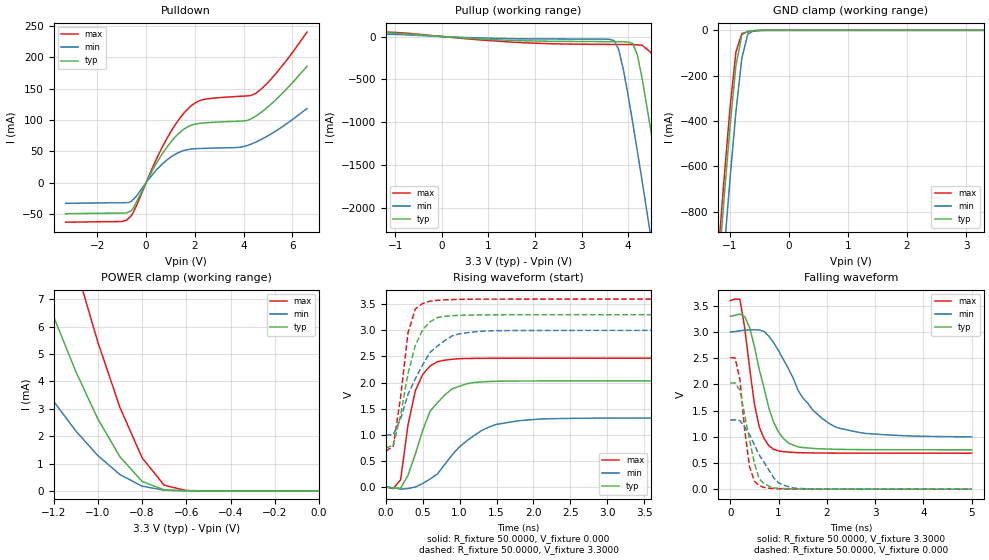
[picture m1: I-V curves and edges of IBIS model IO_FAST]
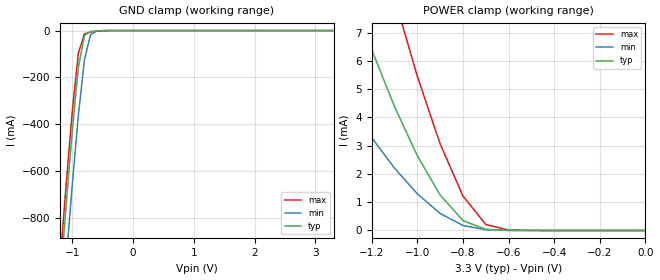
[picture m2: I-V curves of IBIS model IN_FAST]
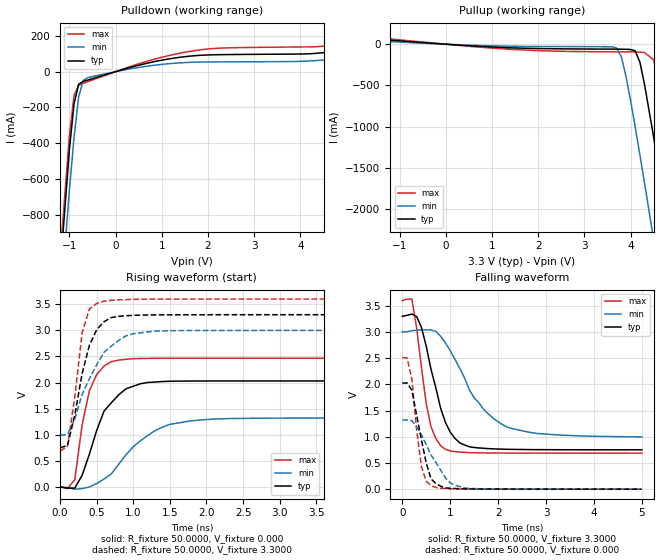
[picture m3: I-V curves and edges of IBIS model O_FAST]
| IBIS file xc4kxl.ibs created by s2ibis2 version 1.1
| North Carolina State University Electronics Research Laboratory  1995
[IBIS ver]   2.1
[File name]   xc4kxl.ibs
[File Rev]   1.5
[Date]   June 18, 2002
[Source]   Hspice simulations (35sTT,SS,FF)
[Notes]   Xilinx IBIS model for XC4kxl (fast slew rate)
   The package models are provided for BG432, BG256, BG352,
   BG560, HQ240, HT144, PQ240, PQ208, PQ160, PQ100, TQ144,
   and VQ100 package types, with BG432 as default. Please make
   your own selection of the packages by commenting out those
   unused ones.
   Control flag setting:
   2 slew rate opts are provided in the model: fast and slow.
   IO_FAST - Input/output Buffer model & fast slew rate
   I_FAST  - Input Buffer model & fast slew rate
   O_FAST  - Output Buffer model & fast slew rate
   IO_SLOW - Input/output Buffer model & slow slew rate
   I_SLOW  - Input Buffer model & slow slew rate
   O_SLOW  - Output Buffer model & slow slew rate
   COMMENTS: Models include process corners for MIN and MAX.
[Disclaimer] The data in this model is derived from SPICE simulations using
   modeling information extracted from the target process. While
   a great deal of care has been taken to provide information
   that is accurate, this model is considered preliminary as it
   has not been verified by actual silicon measurement. Treat the
   data in this model as preliminary until actual silicon
   verification is performed.
[Copyright]   Copyright 2002, Xilinx Inc., All rights reserved
|   Component XC4kxl
|   >>> Make Your Selection of the Package type Below <<<
[Component]   XC4kxl
[Manufacturer]   Xilinx Inc.
[Package]
| For package type BG432
| variable   typ   min   max
R_pkg   0.2500   0.1600   0.3500
L_pkg   4.9000nH   2.4000nH   7.4000nH
C_pkg   1.1500pF   0.8000pF   1.5000pF
| For package type BG256
| variable   typ   min   max
|R_pkg   0.057   0.05   0.065
|L_pkg   4.65nH   3.30nH   6.00nH
|C_pkg   1.05pF   0.80pF   1.30pF
| For package type BG352
| variable   typ   min   max
|R_pkg   0.218   0.145   0.290
|L_pkg   7.20nH   3.40nH   11.0nH
|C_pkg   0.95pF   0.70pF   1.20pF
| For package type BG560
| variable   typ   min   max
|R_pkg   0.24   0.16   0.32
|L_pkg   6.05nH   3.90nH   8.20nH
|C_pkg   1.05pF   0.70pF   1.40pF
| For package type HQ240
| variable   typ   min   max
|R_pkg   0.208   0.202   0.215
|L_pkg   13.2nH   9.00nH   17.3nH
|C_pkg   2.60pF   2.00pF   3.20pF
| For package type HT144
| variable   typ   min   max
|R_pkg   0.115   0.105   0.124
|L_pkg   9.05nH   4.80nH   13.3nH
|C_pkg   0.90pF   0.70pF   1.10pF
| For package type PQ240
| variable   typ   min   max
|R_pkg   0.208   0.205   0.218
|L_pkg   18.9nH   11.9nH   25.8nH
|C_pkg   2.00pF   1.30pF   2.70pF
| For package type PQ208
| variable   typ   min   max
|R_pkg   0.160   0.120   0.200
|L_pkg   18.7nH   10.3nH   27.0nH
|C_pkg   1.80pF   0.70pF   2.90pF
| For package type PQ160
| variable   typ   min   max
|R_pkg   0.195   0.18   0.21
|L_pkg   18.5nH   11.3nH   25.6nH
|C_pkg   2.10pF   1.50pF   2.70pF
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[Pin]  signal_name   model_name   R_pin   L_pin   C_pin
1   IO_FAST   IO_FAST
1I   I_FAST   IN_FAST
1O   O_FAST   O_FAST
2   IO_SLOW   IO_SLOW
2I   I_SLOW   IN_SLOW
2O   O_SLOW   O_SLOW
3   gnd   GND
4   vdd   POWER
| Models and submodels in the file (6): IO_FAST (I/O), IN_FAST (Input), O_FAST (Output), IO_SLOW (I/O), IN_SLOW (Input), O_SLOW (Output)
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|   Model IO_FAST
[Model]   IO_FAST
Model_type   I/O
Polarity   Non-Inverting
Enable   Active-Low
Vmeas =   1.6500V
Vinl =  0.8
Vinh =  2.0
Cref =  50.0000pF
Rref =   1.0000M
Vref =  0.000V
C_comp   7.0000pF   6.0000pF   8.0000pF
[Temperature Range]   27.0000   100.0000   0.000
[Voltage Range]   3.3000V   3.0000V   3.6000V
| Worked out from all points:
|   slope of the pulldown table from 0 to 0.495 V, typ, clamps not added: 13.9 ohm
|   slope of the pullup table from 0 to 0.495 V, typ, clamps not added: 27.1 ohm
|   GND clamp passes 1 mA (typ) near -0.58 V on its own axis
|   POWER clamp passes 1 mA (typ) near -0.87 V on its own axis
|   rising waveform, R_fixture 50.0000, V_fixture 0.000: 20-80 % time 362ps typ, 565ps min, 207ps max; typ from 0 V to 2.03 V
|   rising waveform, R_fixture 50.0000, V_fixture 3.3000: 20-80 % time 245ps typ, 395ps min, 162ps max; typ from 0.751 V to 3.3 V
|   falling waveform, R_fixture 50.0000, V_fixture 3.3000: 20-80 % time 425ps typ, 818ps min, 274ps max; typ from 3.3 V to 0.751 V
|   falling waveform, R_fixture 50.0000, V_fixture 0.000: 20-80 % time 275ps typ, 478ps min, 180ps max; typ from 2.02 V to 0.001 V
[Pulldown]
| voltage   I(typ)   I(min)   I(max)
-3.3V     -49.3mA    -32.8mA    -62.8mA
-800mV    -48.11mA   -31.6mA    -59.6mA
-500mV    -38.84mA   -25.82mA   -45.39mA
300mV     22.39mA    14.76mA    27.1mA
800mV     53.74mA    34.43mA    66.56mA
1.3V      76.97mA    47.48mA    98.21mA
1.7V      88.86mA    52.78mA    117.1mA
2.3V      95.03mA    54.68mA    131.9mA
3.8V      98.02mA    56.26mA    137.5mA
4.5V      106mA      64.68mA    142.4mA
5.3V      131.4mA    81.93mA    172.8mA
6.6V      185.5mA    118.2mA    239.9mA
[Pullup]
| voltage   I(typ)   I(min)   I(max)
-3.3V     63.98mA    45.77mA    74.9mA
3.7V      -59.9mA    -48.13mA   -92.59mA
3.8V      -60.3mA    -155.1mA   -92.88mA
3.9V      -61.55mA   -391.7mA   -93.16mA
4.1V      -81.44mA   -1.009A    -94.6mA
4.2V      -218.1mA   -1.343A    -97.2mA
4.3V      -487mA     -1.684A    -101mA
4.5V      -1.135A    -2.381A    -191.2mA
4.7V      -1.825A    -3.088A    -749.8mA
4.9V      -2.532A    -3.801A    -1.425A
5.1V      -3.246A    -4.519A    -2.126A
6.6V      -8.69A     -9.964A    -7.553A
[GND_clamp]
| voltage   I(typ)   I(min)   I(max)
-3.3V     -8.626A    -8.837A    -8.551A
-1.2V     -1.073A    -1.312A    -987.3mA
-1.1V     -740.8mA   -978.2mA   -654.8mA
-1V       -426mA     -657.1mA   -343.9mA
-900mV    -157.2mA   -360.9mA   -96.62mA
-800mV    -20.77mA   -124.4mA   -14.17mA
-700mV    -3.846mA   -17.61mA   -6.82mA
-600mV    -1.246mA   -1.662mA   -3.283mA
-300mV    -276.3nA   -435.5nA   -2.755uA
3.3V      151.6pA    7.389nA    160.4pA
[POWER_clamp]
| voltage   I(typ)   I(min)   I(max)
-3.3V     75.42mA    47.28mA    100.2mA
-1.5V     13.67mA    7.363mA    21.72mA
-1.4V     11.06mA    5.873mA    18.06mA
-1.3V     8.626mA    4.508mA    14.56mA
-1.2V     6.385mA    3.279mA    11.27mA
-1.1V     4.373mA    2.199mA    8.21mA
-1V       2.636mA    1.293mA    5.443mA
-900mV    1.25mA     599.1uA    3.055mA
-800mV    347.4uA    174.4uA    1.214mA
-700mV    37.68uA    27.06uA    209.3uA
-600mV    2.828uA    3.397uA    13.73uA
0V        151.6pA    186pA      177.1pA
[Ramp]
| variable   typ   min   max
dV/dt_r   1.1778/0.3241n   0.7476/0.5583n   1.4796/0.2068n
dV/dt_f   1.5292/0.3940n   1.2009/0.8182n   1.7477/0.2630n
R_load = 50.0000
[Rising Waveform]
R_fixture = 50.0000
V_fixture = 0.000
| time   V(typ)   V(min)   V(max)
0s        0V         0V         0V
100ps     -22.13mV   -13.9mV    -32.02mV
200ps     -22.59mV   -42.96mV   137.3mV
300ps     222.1mV    -31.55mV   1.186V
400ps     629.5mV    -1.35mV    1.845V
600ps     1.453V     151.4mV    2.316V
700ps     1.614V     249.8mV    2.4V
1ns       1.93V      771.6mV    2.457V
1.5ns     2.025V     1.199V     2.465V
5ns       2.03V      1.32V      2.466V
[Rising Waveform]
R_fixture = 50.0000
V_fixture = 3.3000
V_fixture_min = 3.0000
V_fixture_max = 3.6000
| time   V(typ)   V(min)   V(max)
0s        750.6mV    990.1mV    686.6mV
100ps     794.3mV    1.003V     778mV
200ps     1.376V     1.301V     1.72V
300ps     2.17V      1.772V     2.952V
400ps     2.715V     2.073V     3.411V
500ps     3.013V     2.341V     3.515V
600ps     3.166V     2.58V      3.559V
800ps     3.268V     2.806V     3.583V
1.2ns     3.293V     2.97V      3.596V
5ns       3.299V     2.999V     3.599V
[Falling Waveform]
R_fixture = 50.0000
V_fixture = 3.3000
V_fixture_min = 3.0000
V_fixture_max = 3.6000
| time   V(typ)   V(min)   V(max)
0s        3.3V       3V         3.6V
200ps     3.343V     3.025V     3.627V
400ps     3.087V     3.041V     2.321V
500ps     2.727V     3.043V     1.629V
600ps     2.284V     3.039V     1.188V
900ps     1.275V     2.795V     760.4mV
1.2ns     885.1mV    2.309V     708.3mV
1.5ns     795.3mV    1.745V     695.1mV
2.2ns     760.8mV    1.181V     688.6mV
5ns       751.4mV    998.5mV    687.1mV
[Falling Waveform]
R_fixture = 50.0000
V_fixture = 0.000
| time   V(typ)   V(min)   V(max)
0s        2.025V     1.32V      2.513V
100ps     2.029V     1.323V     2.505V
200ps     1.886V     1.308V     2.095V
300ps     1.408V     1.19V      1.123V
400ps     937.3mV    1.04V      427.3mV
500ps     497.2mV    846.8mV    152.2mV
600ps     195.2mV    651.4mV    68.61mV
1ns       17.14mV    121mV      8.733mV
1.3ns     6.359mV    23.86mV    3.033mV
5ns       508.1uV    961.2uV    304.7uV
|   Model IN_FAST
[Model]   IN_FAST
Model_type   Input
Polarity   Non-Inverting
Vinl  = 0.8000V
Vinh  = 2.0000V
C_comp   7.0000pF   6.0000pF   8.0000pF
[Temperature Range]   27.0000   100.0000   0.000
[Voltage Range]   3.3000V   3.0000V   3.6000V
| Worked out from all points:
|   GND clamp passes 1 mA (typ) near -0.58 V on its own axis
|   POWER clamp passes 1 mA (typ) near -0.87 V on its own axis
[GND_clamp]
| voltage   I(typ)   I(min)   I(max)
-3.3V     -8.626A    -8.837A    -8.551A
-1.2V     -1.073A    -1.312A    -987.3mA
-1.1V     -740.8mA   -978.2mA   -654.8mA
-1V       -426mA     -657.1mA   -343.9mA
-900mV    -157.2mA   -360.9mA   -96.62mA
-800mV    -20.77mA   -124.4mA   -14.17mA
-700mV    -3.846mA   -17.61mA   -6.82mA
-600mV    -1.246mA   -1.662mA   -3.283mA
-300mV    -276.3nA   -435.5nA   -2.755uA
3.3V      151.6pA    7.389nA    160.4pA
[POWER_clamp]
| voltage   I(typ)   I(min)   I(max)
-3.3V     75.42mA    47.28mA    100.2mA
-1.5V     13.67mA    7.363mA    21.72mA
-1.4V     11.06mA    5.873mA    18.06mA
-1.3V     8.626mA    4.508mA    14.56mA
-1.2V     6.385mA    3.279mA    11.27mA
-1.1V     4.373mA    2.199mA    8.21mA
-1V       2.636mA    1.293mA    5.443mA
-900mV    1.25mA     599.1uA    3.055mA
-800mV    347.4uA    174.4uA    1.214mA
-700mV    37.68uA    27.06uA    209.3uA
-600mV    2.828uA    3.397uA    13.73uA
0V        151.6pA    186pA      177pA
|   Model O_FAST
[Model]   O_FAST
Model_type   Output
Polarity   Non-Inverting
Vmeas =   1.6500V
Cref =  50.0000pF
Rref =   1.0000M
Vref =  0.000V
C_comp   7.0000pF   6.0000pF   8.0000pF
[Temperature Range]   27.0000   100.0000   0.000
[Voltage Range]   3.3000V   3.0000V   3.6000V
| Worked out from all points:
|   slope of the pulldown table from 0 to 0.495 V, typ, clamps not added: 13.9 ohm
|   slope of the pullup table from 0 to 0.495 V, typ, clamps not added: 27.1 ohm
|   rising waveform, R_fixture 50.0000, V_fixture 0.000: 20-80 % time 362ps typ, 565ps min, 207ps max; typ from 0 V to 2.03 V
|   rising waveform, R_fixture 50.0000, V_fixture 3.3000: 20-80 % time 245ps typ, 395ps min, 162ps max; typ from 0.751 V to 3.3 V
|   falling waveform, R_fixture 50.0000, V_fixture 3.3000: 20-80 % time 425ps typ, 818ps min, 274ps max; typ from 3.3 V to 0.751 V
|   falling waveform, R_fixture 50.0000, V_fixture 0.000: 20-80 % time 275ps typ, 478ps min, 180ps max; typ from 2.02 V to 0.001 V
[Pulldown]
| voltage   I(typ)   I(min)   I(max)
-3.3V     -8.627A    -8.838A    -8.552A
-1.5V     -2.118A    -2.351A    -2.033A
-1V       -436.6mA   -662mA     -358.9mA
-900mV    -180.8mA   -369.1mA   -134.7mA
-800mV    -70.38mA   -141.6mA   -75.77mA
-700mV    -54.92mA   -48.08mA   -64.92mA
-600mV    -46.83mA   -33mA      -55.57mA
600mV     42.12mA    27.32mA    51.67mA
1.6V      86.5mA     51.89mA    113mA
2.3V      95.03mA    54.68mA    131.9mA
4.5V      106mA      64.68mA    142.4mA
6.6V      185.5mA    118.2mA    239.9mA
[Pullup]
| voltage   I(typ)   I(min)   I(max)
-3.3V     139.4mA    93.05mA    175.1mA
3.7V      -59.9mA    -48.13mA   -92.59mA
3.8V      -60.3mA    -155.1mA   -92.88mA
3.9V      -61.55mA   -391.7mA   -93.16mA
4.1V      -81.44mA   -1.009A    -94.6mA
4.2V      -218.1mA   -1.343A    -97.2mA
4.3V      -487mA     -1.684A    -101mA
4.5V      -1.135A    -2.381A    -191.2mA
4.7V      -1.825A    -3.088A    -749.8mA
4.9V      -2.532A    -3.801A    -1.425A
5.1V      -3.246A    -4.519A    -2.126A
6.6V      -8.69A     -9.964A    -7.553A
[Ramp]
| variable   typ   min   max
dV/dt_r   1.1778/0.3241n   0.7476/0.5583n   1.4796/0.2068n
dV/dt_f   1.5292/0.3940n   1.2009/0.8182n   1.7477/0.2630n
R_load = 50.0000
[Rising Waveform]
R_fixture = 50.0000
V_fixture = 0.000
| time   V(typ)   V(min)   V(max)
0s        0V         0V         0V
100ps     -22.13mV   -13.9mV    -32.02mV
200ps     -22.59mV   -42.96mV   137.3mV
300ps     222.1mV    -31.55mV   1.186V
400ps     629.5mV    -1.35mV    1.845V
600ps     1.453V     151.4mV    2.316V
700ps     1.614V     249.8mV    2.4V
1ns       1.93V      771.6mV    2.457V
1.5ns     2.025V     1.199V     2.465V
5ns       2.03V      1.32V      2.466V
[Rising Waveform]
R_fixture = 50.0000
V_fixture = 3.3000
V_fixture_min = 3.0000
V_fixture_max = 3.6000
| time   V(typ)   V(min)   V(max)
0s        750.6mV    990.1mV    686.6mV
100ps     794.3mV    1.003V     778mV
200ps     1.376V     1.301V     1.72V
300ps     2.17V      1.772V     2.952V
400ps     2.715V     2.073V     3.411V
500ps     3.013V     2.341V     3.515V
600ps     3.166V     2.58V      3.559V
800ps     3.268V     2.806V     3.583V
1.2ns     3.293V     2.97V      3.596V
5ns       3.299V     2.999V     3.599V
[Falling Waveform]
R_fixture = 50.0000
V_fixture = 3.3000
V_fixture_min = 3.0000
V_fixture_max = 3.6000
| time   V(typ)   V(min)   V(max)
0s        3.3V       3V         3.6V
200ps     3.343V     3.025V     3.627V
400ps     3.087V     3.041V     2.321V
500ps     2.727V     3.043V     1.629V
600ps     2.284V     3.039V     1.188V
900ps     1.275V     2.795V     760.4mV
1.2ns     885.1mV    2.309V     708.3mV
1.5ns     795.3mV    1.745V     695.1mV
2.2ns     760.8mV    1.181V     688.6mV
5ns       751.4mV    998.5mV    687.1mV
[Falling Waveform]
R_fixture = 50.0000
V_fixture = 0.000
| time   V(typ)   V(min)   V(max)
0s        2.025V     1.32V      2.513V
100ps     2.029V     1.323V     2.505V
200ps     1.886V     1.308V     2.095V
300ps     1.408V     1.19V      1.123V
400ps     937.3mV    1.04V      427.3mV
500ps     497.2mV    846.8mV    152.2mV
600ps     195.2mV    651.4mV    68.61mV
1ns       17.14mV    121mV      8.733mV
1.3ns     6.359mV    23.86mV    3.033mV
5ns       508.1uV    961.2uV    304.7uV
